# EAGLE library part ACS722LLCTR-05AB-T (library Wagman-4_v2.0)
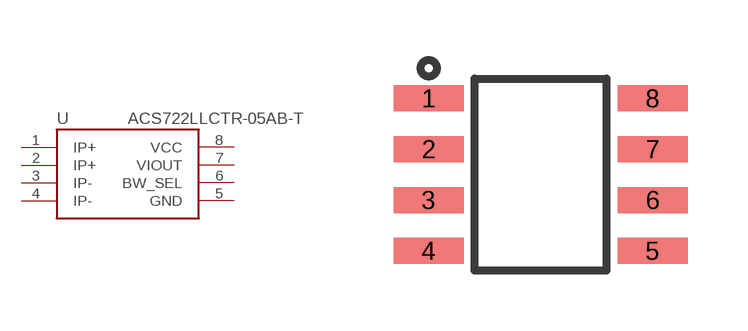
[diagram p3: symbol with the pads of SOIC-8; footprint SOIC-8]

Designator prefix U

## ACS722LLCTR-05AB-T  [SOIC-8]
1  IP+  pas
2  IP+  pas
3  IP-  pas
4  IP-  pas
5  GND  pas
6  BW_SEL  pas
7  VIOUT  pas
8  VCC  pas

## Footprint SOIC-8 (pad centres in mm)
smd 1.75 x 0.65: 1 -2.8,1.905; 2 -2.8,0.635; 3 -2.8,-0.635; 4 -2.8,-1.905; 5 2.8,-1.905; 6 2.8,-0.635; 7 2.8,0.635; 8 2.8,1.905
